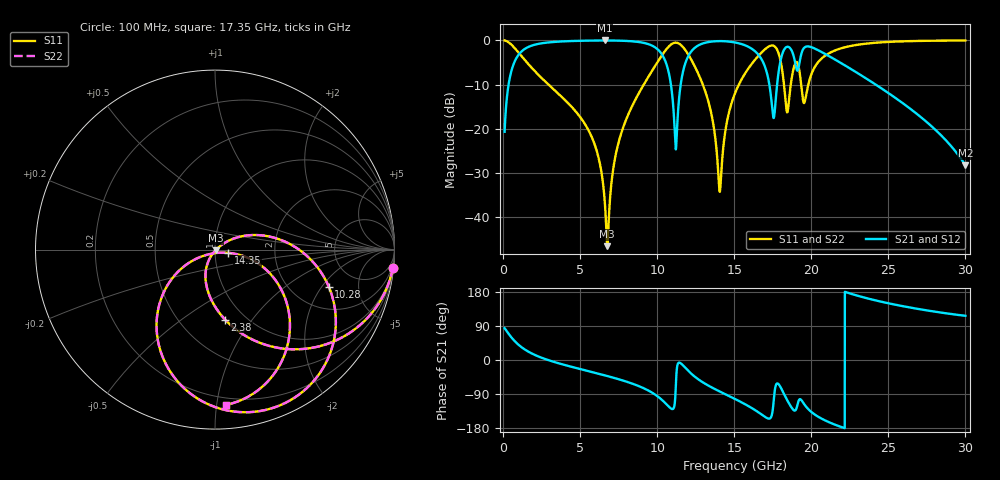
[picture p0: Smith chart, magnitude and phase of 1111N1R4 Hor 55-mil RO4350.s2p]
# GHz S MA R 50
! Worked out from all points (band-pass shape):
!   3201 points, 100 MHz to 30 GHz, reference 50 ohm
!   highest |S21| = -0.05 dB at 6.585 GHz (marker M1); lowest = -28.2 dB at 30 GHz (marker M2)
!   |S21| within 3 dB of the highest: 1.057 GHz to 10.28 GHz (9.225 GHz wide, 163 % of centre); 12.11 GHz to 16.52 GHz (4.411 GHz wide, 30.8 % of centre)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
!   lowest |S11| = -46.5 dB at 6.762 GHz (marker M3), VSWR 1.01, Z = 50.3 - j0.349 ohm
!   |S11| at or under -10 dB: 2.95 GHz to 9.13 GHz (6.18 GHz wide, 102 % of centre); 12.96 GHz to 15.3 GHz (2.339 GHz wide, 16.6 % of centre); 19.34 GHz to 19.81 GHz (464.1 MHz wide, 2.37 % of centre)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
!   |S22| runs from -46.5 to 0.0 dB; largest |S21 - S12| = 0
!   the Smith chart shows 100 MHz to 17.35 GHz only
!   S11 on the Smith chart (normalised r, x): 100 MHz: 1, -19; 2.38 GHz: 0.81, -0.75; 10.28 GHz: 3.14, -2.34; 14.35 GHz: 1.16, -0.04; 17.35 GHz: 0.15, -1.06
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0.1  0.9956 -6.0  0.09285 84.0  0.09285 84.0  0.9956 -6.0
0.7634062  0.8132 -40.5  0.5812 49.5  0.5812 49.5  0.8132 -40.5
2.379875  0.3937 -81.8  0.9172 7.9  0.9172 7.9  0.3937 -81.8
5.089563  0.1297 -113.3  0.9878 -24.8  0.9878 -24.8  0.1297 -113.3
6.584562  0.01624 -114.3  0.9946 -40.4  0.9946 -40.4  0.01624 -114.3
6.762094  0.004742 -47.0  0.9945 -42.3  0.9945 -42.3  0.004742 -47.0
7.64975  0.08725 33.4  0.9891 -52.6  0.9891 -52.6  0.08725 33.4
10.06978  0.5846 -10.3  0.7792 -97.2  0.7792 -97.2  0.5846 -10.3
10.28469  0.6666 -18.0  0.7029 -104.4  0.7029 -104.4  0.6666 -18.0
11.20972  0.9401 -67.7  0.05867 -68.8  0.05867 -68.8  0.9401 -67.7
12.25622  0.5849 -123.3  0.7648 -37.8  0.7648 -37.8  0.5849 -123.3
14.03153  0.02093 -103.6  0.9789 -82.6  0.9789 -82.6  0.02093 -103.6
14.34922  0.07636 -13.6  0.9763 -88.9  0.9763 -88.9  0.07636 -13.6
15.05  0.2519 -17.7  0.945 -102.9  0.945 -102.9  0.2519 -17.7
17.34856  0.8674 -86.1  0.2609 -153.2  0.2609 -153.2  0.8674 -86.1
17.92788  0.6668 -129.3  0.4985 -66.4  0.4985 -66.4  0.6668 -129.3
18.43244  0.1536 -104.3  0.8445 -105.6  0.8445 -105.6  0.1536 -104.3
18.98372  0.5587 -85.5  0.5282 -132.2  0.5282 -132.2  0.5587 -85.5
19.535  0.1957 -87.6  0.8217 -116.2  0.8217 -116.2  0.1957 -87.6
20.03956  0.4283 -58.0  0.8321 -138.3  0.8321 -138.3  0.4283 -58.0
25.01978  0.959 -121.8  0.2527 149.5  0.2527 149.5  0.959 -121.8
30  0.9944 -155.9  0.03881 116.7  0.03881 116.7  0.9944 -155.9
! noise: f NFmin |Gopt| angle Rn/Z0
0.1  0.002253  0.9294  2.685  0.007082
3.417  0.01245  0.5685  24.46  0.004995
6.743  0.0243  0.5703  42.22  0.008994
10.06  0.08259  0.7916  60.22  0.06146
13.39  0.07216  0.7026  80.28  0.0284
16.7  0.1708  0.835  95.75  0.09938
20.03  0.1686  0.8033  112.5  0.05639
23.35  0.1592  0.7821  124.4  0.03435
26.67  0.2963  0.8783  140  0.06363
30  1.017  0.964  156.7  0.2644
